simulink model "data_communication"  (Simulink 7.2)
settings: Solver=FixedStepDiscrete  SolverMode=SingleTasking  StartTime=0  StopTime=30  FixedStep=0.06  RelTol=1e-3
PreLoadFcn:
  | xlsreadsdo('nxtscanner.xls','mpt');
undefined symbols (not defined in the file or in its folder): ScannerBufferInfoEnum

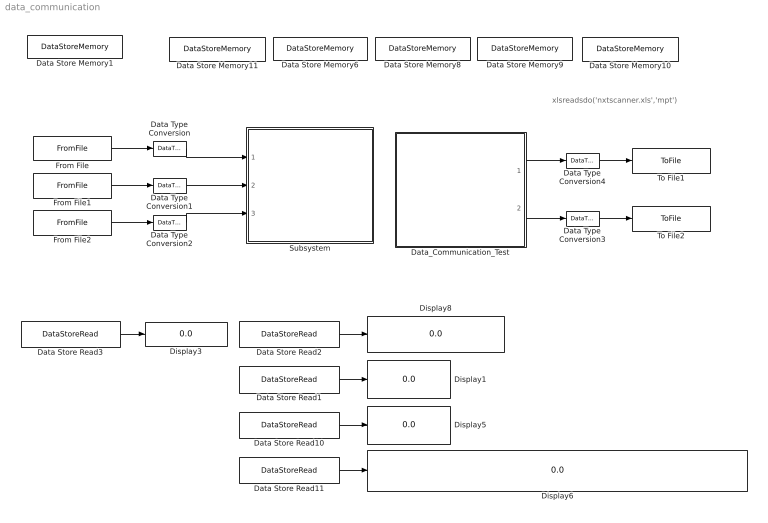
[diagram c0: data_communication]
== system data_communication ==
  note: xlsreadsdo('nxtscanner.xls','mpt')
  Data Store Memory1 : DataStoreMemory  DataStoreName=ErrorCode  ReadBeforeWriteMsg=warning  WriteAfterWriteMsg=warning  WriteAfterReadMsg=warning  InitialValue=ErrorCodeEnum.NO_ERROR  DataType=Specify via dialog  OutDataType=Enum: ErrorCodeEnum  OutDataTypeStr=Enum: ErrorCodeEnum
  Data Store Memory10 : DataStoreMemory  DataStoreName=ScannerBuffer_Pnum  ReadBeforeWriteMsg=warning  WriteAfterWriteMsg=warning  WriteAfterReadMsg=warning  InitialValue=[0;0]  DataType=uint8  OutDataType=Enum: FeedModeEnum  OutDataTypeStr=uint8
  Data Store Memory11 : DataStoreMemory  DataStoreName=ScannerBuffer_Info  ReadBeforeWriteMsg=warning  WriteAfterWriteMsg=warning  WriteAfterReadMsg=warning  InitialValue=[ScannerBufferInfoEnum.TRANS_FINISH;ScannerBufferInfoEnum.TRANS_FINISH]  DataType=Specify via dialog  OutDataType=Enum: ScannerBufferInfoEnum  OutDataTypeStr=Enum: ScannerBufferInfoEnum
  Data Store Memory6 : DataStoreMemory  DataStoreName=ScannerBuffer_Status  ReadBeforeWriteMsg=warning  WriteAfterWriteMsg=warning  WriteAfterReadMsg=warning  InitialValue=[0;0]  DataType=uint16  OutDataType=Enum: ScannerBufferStatusEnum  OutDataTypeStr=uint16
  Data Store Memory8 : DataStoreMemory  DataStoreName=ScannerBuffer_Number  ReadBeforeWriteMsg=warning  WriteAfterWriteMsg=warning  WriteAfterReadMsg=warning  InitialValue=[0;0]  DataType=uint8  OutDataType=Enum: FeedModeEnum  OutDataTypeStr=uint8
  Data Store Memory9 : DataStoreMemory  DataStoreName=ScannerBuffer_Data  ReadBeforeWriteMsg=warning  WriteAfterWriteMsg=warning  WriteAfterReadMsg=warning  InitialValue=[0 0 0 0 0 0 0 0 0 0 0 0 0 0 0 0 0 0 0 0 0 0 0 0 0 0 0 0 0 0; 0 0 0 0 0 0 0 0 0 0 0 0 0 0 0 0 0 0 0 0 0 0 0 0 0 0 0 0 0 0]  DataType=uint16  OutDataType=Enum: FeedModeEnum  OutDataTypeStr=uint16
  Data Store Read1 : DataStoreRead  DataStoreName=ScannerBuffer_Status  SampleTime=0.06
  Data Store Read10 : DataStoreRead  DataStoreName=ScannerBuffer_Number  SampleTime=0.06
  Data Store Read11 : DataStoreRead  DataStoreName=ScannerBuffer_Data  SampleTime=0.06
  Data Store Read2 : DataStoreRead  DataStoreName=ScannerBuffer_Info  SampleTime=0.06
  Data Store Read3 : DataStoreRead  DataStoreName=ErrorCode  SampleTime=0.06
  Data Type Conversion{,1..4} (5 alike) : DataTypeConversion  OutDataType=sfix(16)  OutScaling=2^0
  Data_Communication_Test : Subsystem
  Display{1,3,5..6,8} (5 alike) : Display
  From File : FromFile  FileName=usb_test_state.mat  SampleTime=0.06
  From File1 : FromFile  FileName=usb_test_number.mat  SampleTime=0.06
  From File2 : FromFile  FileName=usb_test_data.mat  SampleTime=0.06
  Subsystem : Subsystem
  To File1 : ToFile  Filename=usb_result.mat  MatrixName=usb_result
  To File2 : ToFile  Filename=usb_result1.mat  MatrixName=usb_result1
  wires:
  Data Store Read3/1 -> Display3/1
  Data Store Read10/1 -> Display5/1
  Data Store Read11/1 -> Display6/1
  Data Store Read2/1 -> Display8/1
  From File/1 -> Data Type Conversion/1
  Data Type Conversion/1 -> Subsystem/1(states)
  From File1/1 -> Data Type Conversion1/1
  Data Type Conversion1/1 -> Subsystem/2(number)
  From File2/1 -> Data Type Conversion2/1
  Data Type Conversion2/1 -> Subsystem/3(data)
  Data Store Read1/1 -> Display1/1
  Data Type Conversion4/1 -> To File1/1
  Data Type Conversion3/1 -> To File2/1
  Data_Communication_Test/1(Out1) -> Data Type Conversion4/1
  Data_Communication_Test/2(Out2) -> Data Type Conversion3/1

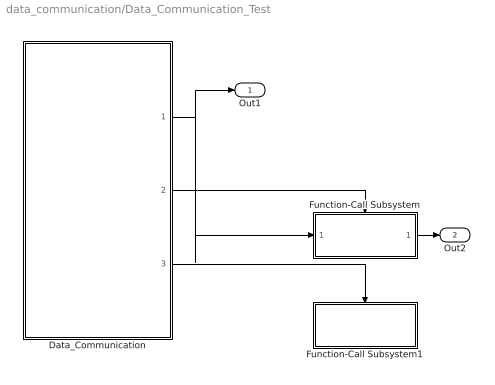
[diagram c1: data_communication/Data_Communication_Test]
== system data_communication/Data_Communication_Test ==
  Data_Communication : Subsystem
  Function-Call Subsystem : Subsystem  TreatAsAtomicUnit=on
  Function-Call Subsystem1 : Subsystem  TreatAsAtomicUnit=on
  Out1 : Outport  OutDataType=sfix(16)  OutScaling=2^0
  Out2 : Outport  Port=2  OutDataType=sfix(16)  OutScaling=2^0
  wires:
  Data_Communication/1(usb_trans_data) -> Out1/1, Function-Call Subsystem/1(In1)
  Data_Communication/2(request_event) -> Function-Call Subsystem/Trigger
  Function-Call Subsystem/1(Out1) -> Out2/1
  Data_Communication/3(disconnect_event) -> Function-Call Subsystem1/Trigger

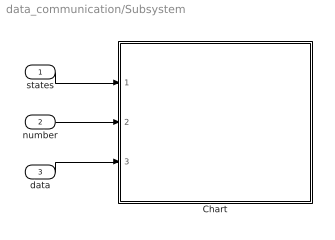
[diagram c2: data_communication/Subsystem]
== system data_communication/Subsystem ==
  states : Inport  OutDataType=sfix(16)  OutScaling=2^0
  number : Inport  Port=2  OutDataType=sfix(16)  OutScaling=2^0
  data : Inport  Port=3  OutDataType=sfix(16)  OutScaling=2^0
  Chart : Stateflow chart
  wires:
  states/1 -> Chart/1(states)
  number/1 -> Chart/2(number)
  data/1 -> Chart/3(data)

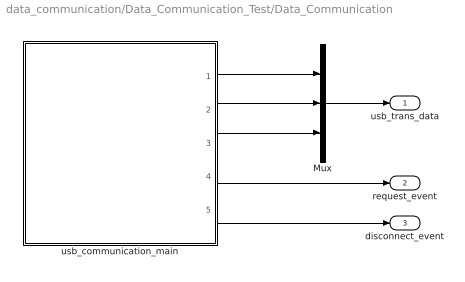
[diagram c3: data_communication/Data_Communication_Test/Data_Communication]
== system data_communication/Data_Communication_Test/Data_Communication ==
  Mux : Mux  Inputs=3
  usb_communication_main : Stateflow chart
  usb_trans_data : Outport  OutDataType=sfix(16)  OutScaling=2^0
  request_event : Outport  Port=2  OutDataType=sfix(16)  OutScaling=2^0
  disconnect_event : Outport  Port=3  OutDataType=sfix(16)  OutScaling=2^0
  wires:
  Mux/1 -> usb_trans_data/1
  usb_communication_main/1(usb_send_status) -> Mux/1
  usb_communication_main/2(usb_send_number) -> Mux/2
  usb_communication_main/3(usb_send_data) -> Mux/3
  usb_communication_main/4(COMUNICATION) -> request_event/1
  usb_communication_main/5(DISCONNECT) -> disconnect_event/1

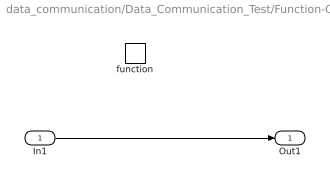
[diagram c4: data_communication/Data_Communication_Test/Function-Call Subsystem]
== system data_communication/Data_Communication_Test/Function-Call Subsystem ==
  In1 : Inport  OutDataType=sfix(16)  OutScaling=2^0
  function : TriggerPort  TriggerType=function-call
  Out1 : Outport  OutDataType=sfix(16)  OutScaling=2^0
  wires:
  In1/1 -> Out1/1

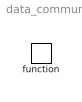
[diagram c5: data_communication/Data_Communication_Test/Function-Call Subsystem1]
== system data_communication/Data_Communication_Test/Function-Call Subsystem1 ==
  function : TriggerPort  TriggerType=function-call

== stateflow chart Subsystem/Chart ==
  state data_generate(a) [function]
    (junction 6) -> (junction 8) : { ScannerBuffer_Info[a] = FULL_UP; ScannerBuffer_Status[a] = 0x0; ScannerBuffer_Number[a] = number; }
    (default) -> (junction 6)
    (junction 7) -> (junction 10) : [index < 30]
    (junction 10) -> (junction 11) : { ScannerBuffer_Data[a][index] = data[index]; }
    (junction 11) -> (junction 7) : { index++; }
    (junction 7) -> (junction 12)
    (junction 8) -> (junction 7) : { index = 0; }
  state data_refresh(k) [function]
    (default) -> (junction 20)
    (junction 20) -> (junction 21) : { ScannerBuffer_Status[k] = STORING; ScannerBuffer_Number[k] = 0; }
    (junction 21) -> (junction 23) : { index = 0; }
    (junction 23) -> (junction 22) : [index < 30]
    (junction 22) -> (junction 24) : { ScannerBuffer_Data[k][index] = 0; }
    (junction 24) -> (junction 23) : { index++; }
    (junction 23) -> (junction 17)
  (default) -> (junction 5)
  (junction 15) -> (junction 25) : { cnt++; }
  (junction 14) -> (junction 15)
  (junction 5) -> (junction 13) : [cnt%%10 == 0]
  (junction 9) -> (junction 14) : { data_generate(select); }
  (junction 5) -> (junction 15) : { data_refresh(0); data_refresh(1); }
  (junction 13) -> (junction 18) : { data_refresh(select); }
  (junction 18) -> (junction 16) : [select == 0]
  (junction 16) -> (junction 19) : { select = 1; }
  (junction 19) -> (junction 9)
  (junction 18) -> (junction 9) : { select = 0; }

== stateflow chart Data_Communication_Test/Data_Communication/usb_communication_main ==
  state usb_communication(arg_select_buffer) [function]
    (junction 85) -> (junction 81)
    (default) -> (junction 83) : { %status high 8 bits is zero usb_send_status[1] = 0; usb_send_status[0] = ScannerBuffer_Status[arg_select_buffer]; %number high 8 bits is zero usb_send_number[1] = 0; usb_send_number[0] = ScannerBuffer_Number[arg_select_buffer]; }
    (junction 83) -> (junction 85) : { index = 0; }
    (junction 85) -> (junction 84) : [index < 30]
    (junction 84) -> (junction 74) : { % split data uint16 to uint8 usb_send_data[index*2+1] = (ScannerBuffer_Data[arg_select_buffer][index] & 0xFF00) >> 8; usb_send_data[index*2] = ScannerBuffer_Data[arg_select_buffer][index] & 0x00FF; }
    (junction 74) -> (junction 85) : { index++; }
  state init_buffer(arg_select_buf) [function]
    (junction 73) -> (junction 71)
    (junction 78) -> (junction 72) : { ScannerBuffer_Data[arg_select_buf][index] = 0; }
    (junction 75) -> (junction 76) : { ScannerBuffer_Info[arg_select_buf] = TRANS_FINISH; ScannerBuffer_Status[arg_select_buf] = 0; ScannerBuffer_Number[arg_select_buf] = 0; ScannerBuffer_Pnum[arg_select_buf] = 0; }
    (junction 72) -> (junction 73) : { index++; }
    (junction 76) -> (junction 73) : { index = 0; }
    (junction 73) -> (junction 78) : [index < 30]
    (default) -> (junction 75)
  state final = usb_final_check [function]
    (junction 82) -> (junction 79) : [(usb_send_status[0] & 0x15) == 0x15]
    (junction 80) -> (junction 77)
    (junction 79) -> (junction 80) : { final = 1; }
    (junction 82) -> (junction 77) : { final = 0; }
    (default) -> (junction 82) : { % VALID(bit0) STOP(bit2) ELP(bit4) check }
  state CLOSE/
    en:
    DISCONNECT;
    disconnect = 0;
  state OPEN/
    en:
    usb_function();
    disconnect = usb_final_check();
    du:
    usb_function();
    disconnect = usb_final_check();
  state usb_function [function]
    (default) -> (junction 91) : { usb_send_status = 0; usb_send_number = 0; usb_send_data = 0; disconnect = 0; }
    (junction 87) -> (junction 89)
    (junction 87) -> (junction 88) : [ScannerBuffer_Info[0] == FULL_UP]
    (junction 89) -> (junction 86) : { % nothing }
    (junction 88) -> (junction 98) : { % USB sending usb_communication(0); init_buffer(0); COMUNICATION; }
    (junction 89) -> (junction 90) : [ScannerBuffer_Info[1] == FULL_UP]
    (junction 90) -> (junction 97) : { % USB sending usb_communication(1); init_buffer(1); COMUNICATION; }
    (junction 94) -> (junction 93) : [ ScannerBuffer_Pnum[0] <= ScannerBuffer_Pnum[1] ]
    (junction 91) -> (junction 87)
    (junction 91) -> (junction 92) : [ScannerBuffer_Info[0] == FULL_UP && ScannerBuffer_Info[1] == FULL_UP]
    (junction 93) -> (junction 95) : { % USB sending usb_communication(0); init_buffer(0); COMUNICATION; }
    (junction 94) -> (junction 96) : { % USB sending usb_communication(1); init_buffer(1); COMUNICATION; }
    (junction 92) -> (junction 94)
    (junction 95) -> (junction 96)
    (junction 96) -> (junction 98)
    (junction 98) -> (junction 97)
    (junction 97) -> (junction 86)
  (default) -> OPEN
  OPEN -> CLOSE : [disconnect == 1]
  CLOSE -> OPEN : [disconnect == 0]
